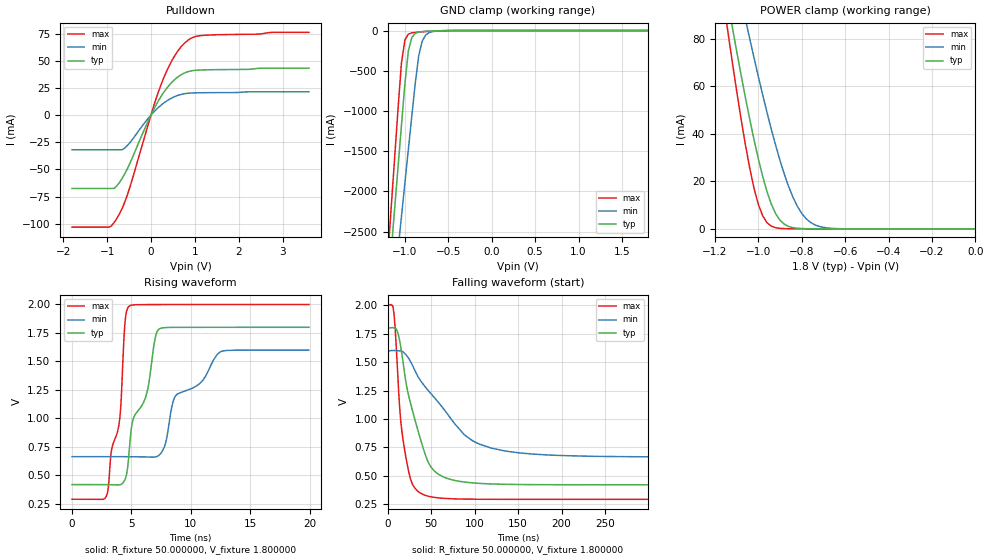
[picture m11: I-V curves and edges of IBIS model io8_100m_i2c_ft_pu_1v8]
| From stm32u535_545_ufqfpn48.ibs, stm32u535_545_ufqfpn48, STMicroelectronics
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|   Model io8_100m_i2c_ft_pu_1v8
[Model]  io8_100m_i2c_ft_pu_1v8
Model_type I/O_open_drain
Polarity   Non-Inverting
Enable   Active-Low
Vinl =   0.540000V
Vinh =   1.260000V
Vmeas =  0.900000V
Cref =   50.000000pF
Rref =   100.000000M
Vref =   0.900000V
C_comp   3.154800pF   3.154000pF   3.203200pF
[Temperature Range]   25.000000   0.140000k   -40.000000
[Pullup Reference]   1.800000V   1.600000V   2.000000V
[Pulldown Reference]   0.0V   0.0V   0.0V
[POWER Clamp Reference]   1.800000V   1.600000V   2.000000V
[GND Clamp Reference]   0.0V   0.0V   0.0V
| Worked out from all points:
|   slope of the pulldown table from 0 to 0.27 V, typ, clamps not added: 13.8 ohm
|   GND clamp passes 1 mA (typ) near -0.51 V on its own axis
|   POWER clamp passes 1 mA (typ) near -0.86 V on its own axis
|   rising waveform, R_fixture 50.000000, V_fixture 1.800000: 20-80 % time 1.94ns typ, 3.43ns min, 1.12ns max; typ from 0.42 V to 1.8 V
|   falling waveform, R_fixture 50.000000, V_fixture 1.800000: 20-80 % time 25.6ns typ, 57.5ns min, 11.9ns max; typ from 1.8 V to 0.42 V
[Pulldown]
|Voltage   I(typ)   I(min)   I(max)
-1.8V     -67.53mA   -31.92mA   -103.1mA
-960mV    -67.53mA   -31.92mA   -103.1mA
-840mV    -67.53mA   -31.92mA   -98.86mA
-780mV    -65.26mA   -31.92mA   -95.24mA
-660mV    -58.47mA   -31.92mA   -86.15mA
-540mV    -49.6mA    -28.16mA   -73.74mA
0V        0A         0A         0A
240mV     17.82mA    9.483mA    29.05mA
540mV     32.64mA    16.95mA    54.49mA
840mV     39.89mA    20.07mA    68.75mA
1.26V     41.64mA    20.58mA    73.52mA
3.6V      43.13mA    21.42mA    76.15mA
[GND_clamp]
|Voltage   I(typ)   I(min)   I(max)
-1.8V     -9.707A    -9.942A    -9.774A
-1.2V     -3.309A    -4.006A    -2.864A
-1.16V    -2.777A    -3.584A    -2.239A
-1.12V    -2.246A    -3.162A    -1.614A
-1.04V    -1.186A    -2.319A    -408.6mA
-1V       -663.9mA   -1.898A    -117.8mA
-960mV    -254mA     -1.478A    -45.14mA
-920mV    -86.03mA   -1.06A     -28.58mA
-840mV    -19.12mA   -308.9mA   -18.74mA
-800mV    -13.39mA   -130.8mA   -15.31mA
-720mV    -7.948mA   -25.37mA   -9.381mA
1.8V      0A         14.97nA    0A
[POWER_clamp]
|Voltage   I(typ)   I(min)   I(max)
-1.8V     470.9mA    433.7mA    554.6mA
-1.14V    95.28mA    122.7mA    82.88mA
-1.12V    85mA       114mA      70.34mA
-1.06V    55.55mA    88.43mA    35.73mA
-1.04V    46.38mA    80.17mA    25.83mA
-1V       29.54mA    64.14mA    10.37mA
-940mV    10.43mA    41.88mA    1.177mA
-900mV    3.66mA     28.79mA    250.6uA
-840mV    527.3uA    13.26mA    95.88uA
-800mV    153.9uA    6.55mA     88.57uA
-740mV    60.03uA    1.742mA    70.75uA
0V        0A         18.15nA    0A
[Ramp]
| variable   typ   min   max
dV/dt_r  0.82823/1.93977n   0.56111/3.43273n   1.02529/1.12023n
dV/dt_f  0.82829/25.56062n   0.56116/57.41930n   1.02529/11.92191n
R_load = 50.000000
[Rising Waveform]
R_fixture= 50.000000
V_fixture= 1.800000
V_fixture_min= 1.600000
V_fixture_max= 2.000000
|time   V(typ)   V(min)   V(max)
0s        419.5mV    664.6mV    291.2mV
2.963ns   419mV      664.6mV    337.9mV
3.323ns   418.7mV    664.6mV    720.9mV
4.004ns   417.5mV    664.6mV    984.7mV
4.444ns   460.2mV    664.4mV    1.818V
4.805ns   702mV      664.1mV    1.984V
7.327ns   1.784V     677.5mV    1.999V
8.689ns   1.799V     1.193V     2V
12.45ns   1.8V       1.583V     2V
19.94ns   1.8V       1.6V       2V
[Falling Waveform]
R_fixture= 50.000000
V_fixture= 1.800000
V_fixture_min= 1.600000
V_fixture_max= 2.000000
|time   V(typ)   V(min)   V(max)
0s        1.8V       1.6V       2V
7.207ns   1.801V     1.602V     1.942V
14.41ns   1.671V     1.6V       1.054V
20.82ns   1.34V      1.569V     675.5mV
28.83ns   1.069V     1.47V      421.7mV
38.44ns   806.6mV    1.332V     343.5mV
58.46ns   512.2mV    1.146V     304.2mV
88.89ns   443.2mV    856.6mV    293.3mV
119.3ns   426.9mV    742.7mV    291.6mV
398.8ns   419.5mV    664.6mV    291.2mV
